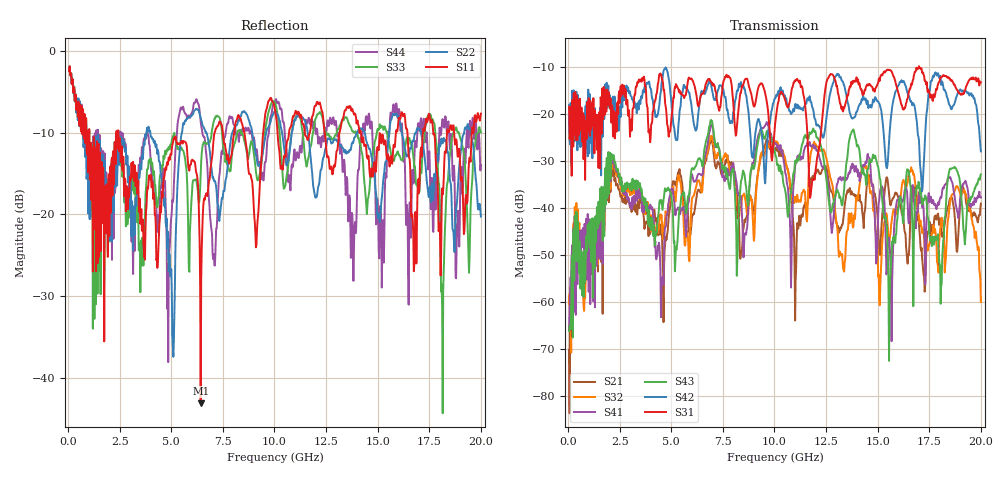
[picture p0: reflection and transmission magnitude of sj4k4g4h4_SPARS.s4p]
! FILE: E:\users\goganessyan\GBX_Backplane\FR408_backplane\1m_OUTBOUND_NEXT\sj4k4g4h4_SPARS.s4p
# MHZ S RI R 50.00
! FREQ  S11  S12  S13  S14
!  S21  S22  S23  S24
!  S31  S32  S33  S34
!  S41  S42  S43  S44
!  REAL  IMAG  REAL  IMAG  REAL  IMAG  REAL  IMAG
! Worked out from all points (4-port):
!   799 points, 50 MHz to 20 GHz, reference 50 ohm
!   strongest paths, dB at 50 MHz, 5.025 GHz, 10.03 GHz, 15.03 GHz, 20 GHz:
!     S31: -18.5, -20.2, -22.4, -13.4, -13.3
!     S42: -18.2, -19.0, -16.7, -17.4, -28.0
!     S43: -66.3, -38.6, -28.2, -31.3, -32.9
!     S41: -66.1, -36.0, -26.3, -41.6, -37.8
!     S32: -60.5, -36.3, -25.8, -54.7, -60.1
!     S21: -70.2, -36.0, -27.7, -44.6, -39.1
!   lowest |S11| = -43.1 dB at 6.425 GHz (marker M1), VSWR 1.01, Z = 49.6 + j0.559 ohm
!   |S11| at or under -10 dB: 1.027 GHz to 2.343 GHz (1.316 GHz wide, 78.1 % of centre); 2.43 GHz to 7.099 GHz (4.67 GHz wide, 98 % of centre); 14.19 GHz to 15.89 GHz (1.701 GHz wide, 11.3 % of centre)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
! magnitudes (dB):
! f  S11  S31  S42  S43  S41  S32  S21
! 50 MHz  -2.5  -18.5  -18.2  -66.3  -66.1  -60.5  -70.2
! 2.175 GHz  -12.3  -24.8  -16.4  -29.1  -30.4  -30.8  -33.2
! 4.55 GHz  -17.3  -12.8  -12.9  -39.6  -55.5  -43.4  -45.9
! 6.425 GHz  -43.1  -16.3  -16.1  -29.9  -33.0  -35.6  -36.8
! 13.8 GHz  -7.4  -13.0  -21.0  -23.5  -31.2  -44.2  -37.1
! 15.57 GHz  -14.2  -10.7  -24.3  -59.1  -47.9  -47.2  -38.2
! 20 GHz  -7.7  -13.3  -28.0  -32.9  -37.8  -60.1  -39.1
